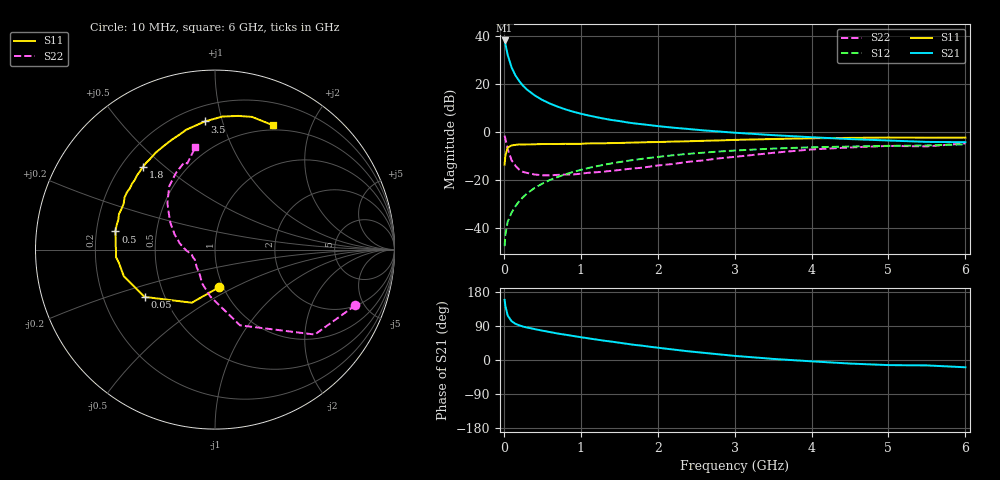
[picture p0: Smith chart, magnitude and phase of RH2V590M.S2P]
! SIEMENS Small Signal Semiconductors
! BFR106
! Si NPN RF Bipolar Junction Transistor in SOT23
! VCE = 2.5 V  IC = 90 mA
! Common Emitter S-Parameters:  August  1996
# GHz  S  MA  R  50
!  f  S11  S21  S12  S22
! GHz  MAG  ANG  MAG  ANG  MAG  ANG  MAG  ANG
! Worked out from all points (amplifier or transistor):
!   36 points, 10 MHz to 6 GHz, reference 50 ohm
!   highest |S21| = 38.0 dB at 10 MHz (marker M1)
!   |S21| within 3 dB of that: start of sweep to 30.32 MHz
!   unconditionally stable (mu >= 1): 152.5 MHz to 2.812 GHz; 5.071 GHz to end of sweep
!   at 250 MHz: K = 1.07, MAG = 21.5 dB, |S12| = -27.0 dB
!   at 1.4 GHz: K = 1.07, MAG = 7.4 dB, |S12| = -13.0 dB
!   at 6 GHz: K = 1.01, MAG = -0.2 dB, |S12| = -5.1 dB
!   S11 on the Smith chart (normalised r, x): 10 MHz: 0.96, -0.42; 50 MHz: 0.39, -0.26; 500 MHz: 0.28, +0.08; 1.8 GHz: 0.29, +0.43; 3.5 GHz: 0.30, +0.88; 6 GHz: 0.44, +1.48
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0.01  0.2111 -83.9  79.16 158.7  0.0043 78.0  0.8419 -21.6
0.02  0.3229 -113.6  67.11 142.8  0.0074 67.4  0.7301 -40.4
0.05  0.4726 -146.1  39.75 117.4  0.0138 61.4  0.4444 -71.7
0.1  0.5293 -163.7  22 102.5  0.0212 65.6  0.2617 -96.0
0.15  0.5403 -172.1  14.99 95.6  0.0288 68.7  0.2004 -111.2
0.2  0.5533 -175.7  11.39 91.4  0.0369 71.5  0.1663 -120.2
0.25  0.5514 -179.3  9.1 88.2  0.0447 72.9  0.1489 -129.6
0.3  0.5533 178.1  7.617 85.8  0.053 73.6  0.1424 -135.2
0.4  0.5568 173.5  5.761 81.6  0.0693 73.5  0.1316 -145.0
0.5  0.5641 169.7  4.631 77.5  0.0851 73.1  0.1268 -151.7
0.6  0.5645 166.0  3.881 73.7  0.1015 72.1  0.1265 -155.5
0.7  0.5639 162.8  3.355 69.9  0.1171 71.0  0.1294 -159.3
0.9  0.5682 156.4  2.644 63.4  0.1488 68.1  0.1318 -166.5
1.1  0.5816 150.1  2.205 57.1  0.1796 65.1  0.143 -170.4
1.4  0.5901 141.6  1.778 48.5  0.2236 60.0  0.157 -177.3
1.8  0.6115 130.9  1.448 37.7  0.2786 53.3  0.1821 173.5
2.2  0.6334 121.3  1.23 27.7  0.3299 46.5  0.2177 164.2
2.8  0.6694 107.4  1.025 14.9  0.3944 36.5  0.2849 150.0
3.5  0.7163 94.5  0.862 2.9  0.4541 25.5  0.3704 135.7
4.5  0.7561 80.1  0.714 -9.4  0.5007 11.1  0.479 117.1
5.5  0.7633 68.9  0.624 -14.3  0.5273 2.3  0.5041 107.8
6  0.7648 64.8  0.616 -19.2  0.5553 -4.6  0.5807 100.9
